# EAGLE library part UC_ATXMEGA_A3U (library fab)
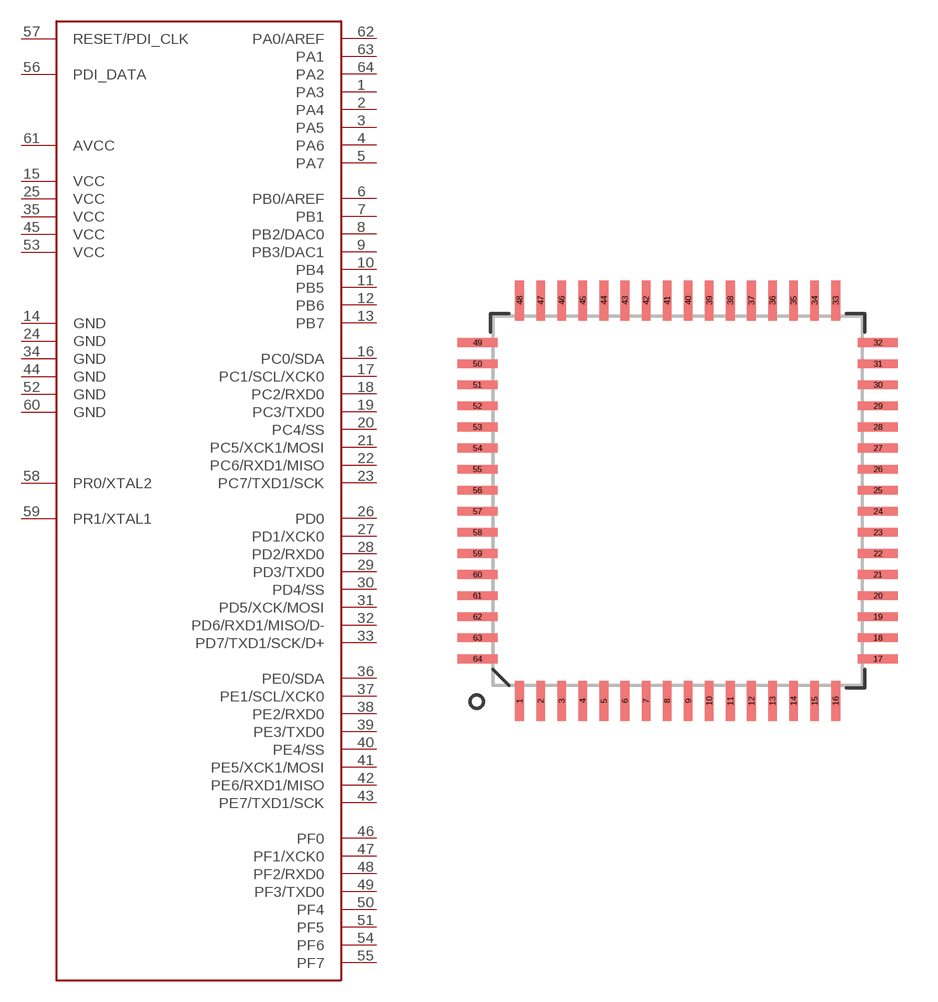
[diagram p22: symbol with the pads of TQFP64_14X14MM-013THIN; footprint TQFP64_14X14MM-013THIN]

Designator prefix -

## UC_ATXMEGA_A3U  [TQFP64_14X14MM-013THIN]
1  PA3
2  PA4
3  PA5
4  PA6
5  PA7
6  PB0/AREF
7  PB1
8  PB2/DAC0
9  PB3/DAC1
10  PB4
11  PB5
12  PB6
13  PB7
14  GND
15  VCC
16  PC0/SDA
17  PC1/SCL/XCK0
18  PC2/RXD0
19  PC3/TXD0
20  PC4/SS
21  PC5/XCK1/MOSI
22  PC6/RXD1/MISO
23  PC7/TXD1/SCK
24  GND
25  VCC
26  PD0
27  PD1/XCK0
28  PD2/RXD0
29  PD3/TXD0
30  PD4/SS
31  PD5/XCK/MOSI
32  PD6/RXD1/MISO/D-
33  PD7/TXD1/SCK/D+
34  GND
35  VCC
36  PE0/SDA
37  PE1/SCL/XCK0
38  PE2/RXD0
39  PE3/TXD0
40  PE4/SS
41  PE5/XCK1/MOSI
42  PE6/RXD1/MISO
43  PE7/TXD1/SCK
44  GND
45  VCC
46  PF0
47  PF1/XCK0
48  PF2/RXD0
49  PF3/TXD0
50  PF4
51  PF5
52  GND
53  VCC
54  PF6
55  PF7
56  PDI_DATA
57  RESET/PDI_CLK
58  PR0/XTAL2
59  PR1/XTAL1
60  GND
61  AVCC
62  PA0/AREF
63  PA1
64  PA2

## Footprint TQFP64_14X14MM-013THIN (pad centres in mm)
64-Lead TQFP Plastic Thin Quad Flatpack - 14x14x1mm Body
smd 0.33 x 1.524: 1 -6,-7.6; 2 -5.2,-7.6; 3 -4.4,-7.6; 4 -3.6,-7.6; 5 -2.8,-7.6; 6 -2,-7.6; 7 -1.2,-7.6; 8 -0.4,-7.6; 9 0.4,-7.6; 10 1.2,-7.6; 11 2,-7.6; 12 2.8,-7.6; 13 3.6,-7.6; 14 4.4,-7.6; 15 5.2,-7.6; 16 6,-7.6; 33 6,7.6; 34 5.2,7.6; 35 4.4,7.6; 36 3.6,7.6; 37 2.8,7.6; 38 2,7.6; 39 1.2,7.6; 40 0.4,7.6; 41 -0.4,7.6; 42 -1.2,7.6; 43 -2,7.6; 44 -2.8,7.6; 45 -3.6,7.6; 46 -4.4,7.6; 47 -5.2,7.6; 48 -6,7.6
smd 1.524 x 0.33: 17 7.6,-6; 18 7.6,-5.2; 19 7.6,-4.4; 20 7.6,-3.6; 21 7.6,-2.8; 22 7.6,-2; 23 7.6,-1.2; 24 7.6,-0.4; 25 7.6,0.4; 26 7.6,1.2; 27 7.6,2; 28 7.6,2.8; 29 7.6,3.6; 30 7.6,4.4; 31 7.6,5.2; 32 7.6,6; 49 -7.6,6; 50 -7.6,5.2; 51 -7.6,4.4; 52 -7.6,3.6; 53 -7.6,2.8; 54 -7.6,2; 55 -7.6,1.2; 56 -7.6,0.4; 57 -7.6,-0.4; 58 -7.6,-1.2; 59 -7.6,-2; 60 -7.6,-2.8; 61 -7.6,-3.6; 62 -7.6,-4.4; 63 -7.6,-5.2; 64 -7.6,-6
